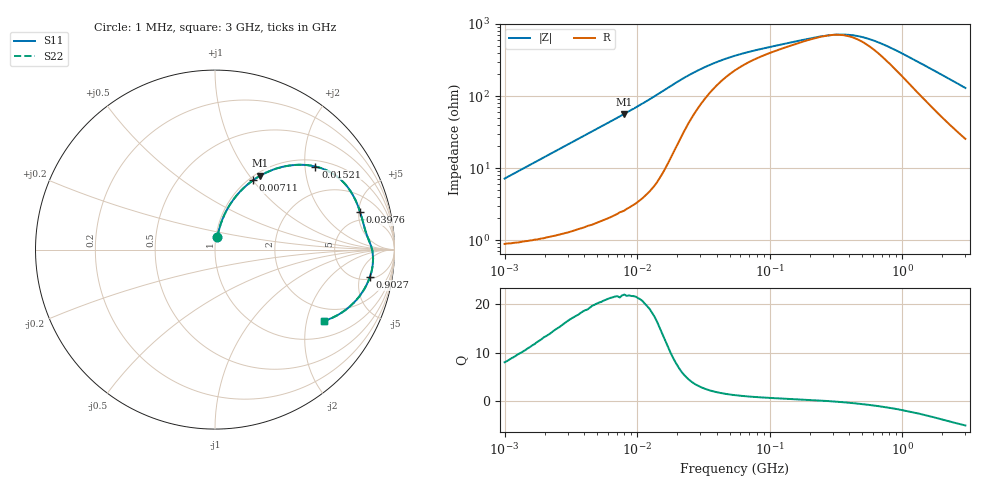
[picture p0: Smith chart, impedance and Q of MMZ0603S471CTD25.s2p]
! S-Parameter Data Generated by TDK Corporation
! Copyright(C) 2025 TDK Corporation.
! All Rights Reserved.
! TDK P/N: MMZ0603S471CTD25 (Chip Bead)
! Property: |Z|=470ohm at 100MHz
! Size(LxWxT): 0.6x0.3x0.3mm
! Model Type: s2p (Touchstone File Format Version 1.0)
! Frequency: DC=Yes Start=1MHz Stop=3000MHz 202points Log-sweep
! Model Generated on Feb. 6, 2025
! Terms and conditions regarding TDK Simulation Models:
! 1)This simulation model is being provided solely for informational
!  purposes. Please refer to the specifications of the products in
!  terms of detailed characteristics of such products.
! 2)In no event shall TDK Corporation of any of its subsidiaries be
!  liable for any loss or damage arising, directly or indirectly,
!  from any information contained in this simulation model, including,
!  but not limited to loss or damages arising from any inaccuracies,
!  omissions or errors in connection with such information.
! 3)Any and all copyrights on this simulation model are owned by
!  TDK Corporation.  Duplication or redistribution of this simulation
!  model without prior written permission from TDK Corporation
!  is prohibited.
! 4)This simulation model is subject to any modification or change
!  without any prior notice.
! 5)Neither TDK Corporation nor any of its subsidiaries shall make any
!  warranty, express or implied, including but not limited to the
!  correctness, implied warranties of merchantability and fitness for
!  a particular purpose with respect to this simulation models.
! 6)The use of this simulation model shall be deemed to have consented
!  to the terms and conditions hereof.
! Port Assignments:
!  1 ---@@@--- 2
! Applicable Conditions:
!  Temperature = 25 degC
!  DC Bias Current = 0 A
!  Small Signal Operation
# Hz S MA R 50
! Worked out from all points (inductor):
!   201 points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, 1 MHz to 3 GHz, reference 50 ohm
!   read as one part in series: L = 1.13 uH near 1.041 MHz
!   highest Q = 21.8 at 8.018 MHz (marker M1), where L = 1.12 uH
!   self-resonance near 287.4 MHz
!   S11 on the Smith chart (normalised r, x): 1 MHz: 1.02, +0.14; 7.11 MHz: 1.05, +1.00; 15.21 MHz: 1.16, +2.27; 39.76 MHz: 3.80, +5.22; 902.7 MHz: 5.56, -7.28; 3 GHz: 1.51, -2.54
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1000000  0.07087 78.9  0.9888 -4.0  0.9888 -4.0  0.07087 78.9
2055611  0.1428 77.5  0.9792 -8.2  0.9792 -8.2  0.1428 77.5
3900413  0.2616 71.8  0.9512 -15.1  0.9512 -15.1  0.2616 71.8
5372736  0.3481 66.9  0.9206 -20.3  0.9206 -20.3  0.3481 66.9
7110411  0.4404 61.2  0.8777 -26.1  0.8777 -26.1  0.4404 61.2
8017732  0.4837 58.5  0.8535 -28.9  0.8535 -28.9  0.4837 58.5
1.104425e7  0.6073 49.9  0.7655 -37.3  0.7655 -37.3  0.6073 49.9
1.461624e7  0.713 40.9  0.6566 -45.4  0.6566 -45.4  0.713 40.9
1.521322e7  0.7264 39.6  0.6386 -46.4  0.6386 -46.4  0.7264 39.6
1.934349e7  0.7898 31.4  0.5246 -51.6  0.5246 -51.6  0.7898 31.4
2.362996e7  0.8169 25.3  0.4355 -53.2  0.4355 -53.2  0.8169 25.3
3.976269e7  0.8352 14.4  0.2821 -47.4  0.2821 -47.4  0.8352 14.4
5.477226e7  0.839 10.4  0.2308 -40.8  0.2308 -40.8  0.839 10.4
2.136344e8  0.8682 1.7  0.1347 -11.0  0.1347 -11.0  0.8682 1.7
3.188066e8  0.8775 -0.7  0.123 4.7  0.123 4.7  0.8775 -0.7
4.219165e8  0.8815 -2.6  0.1258 18.3  0.1258 18.3  0.8815 -2.6
5.81181e8  0.8827 -5.2  0.1452 33.6  0.1452 33.6  0.8827 -5.2
8.005644e8  0.8795 -8.5  0.1841 45.0  0.1841 45.0  0.8795 -8.5
9.0272e8  0.8765 -10.0  0.2041 48.0  0.2041 48.0  0.8765 -10.0
1.712864e9  0.8321 -20.3  0.3621 52.7  0.3621 52.7  0.8321 -20.3
2.266846e9  0.7895 -26.3  0.4558 50.1  0.4558 50.1  0.7895 -26.3
3e9  0.7255 -33.3  0.5602 45.3  0.5602 45.3  0.7255 -33.3
